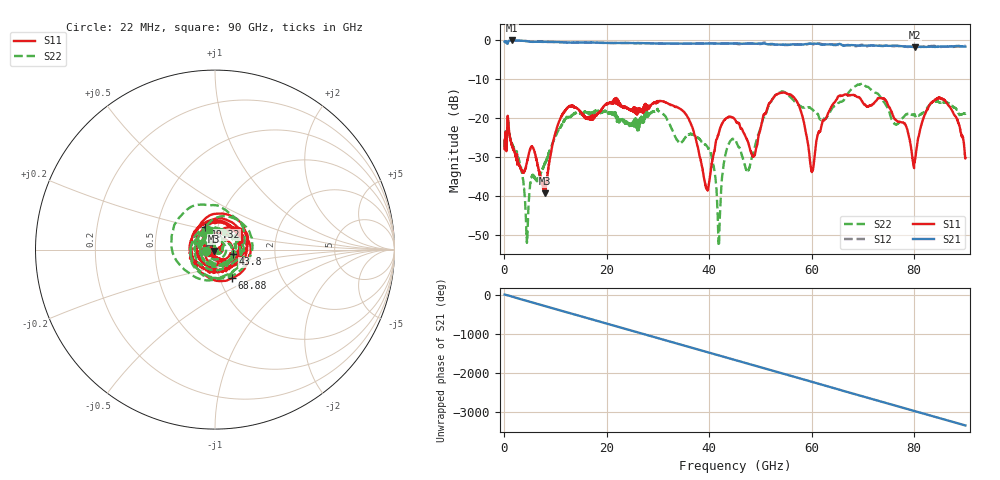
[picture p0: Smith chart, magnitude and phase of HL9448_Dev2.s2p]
! 5/9/2022 12:37:12 PM
! C:\USERS\VECTORSTARUSER\DESKTOP\JASON\HL9449-11\HL9449-11-NE04.S2P
! CHANNEL.1
! TR.MEASUREMENT
! CORRECTED.DATA
# GHZ S RI R 50.0
! FREQ.GHZ  S11RE  S11IM  S21RE  S21IM  S12RE  S12IM  S22RE  S22IM
!; PortSelection: Port_12
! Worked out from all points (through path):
!   4091 points, 22 MHz to 90 GHz, reference 50 ohm
!   highest |S21| = -0.24 dB at 1.386 GHz (marker M1); lowest = -2.0 dB at 80.15 GHz (marker M2)
!   group delay of S21, straight-line fit = 103 ps
!   lowest |S11| = -39.3 dB at 7.942 GHz (marker M3), VSWR 1.02, Z = 49.2 - j0.693 ohm
!   |S11| at or under -10 dB: start of sweep to end of sweep
!   |S22| runs from -52.9 to -11.3 dB; largest |S21 - S12| = 0.038
!   S11 on the Smith chart (normalised r, x): 22 MHz: 0.90, -0.02; 19.32 GHz: 0.87, +0.22; 43.8 GHz: 1.22, -0.06; 68.88 GHz: 1.14, -0.38; 90 GHz: 0.96, -0.04
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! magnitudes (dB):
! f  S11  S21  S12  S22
! 22 MHz  -25.7  -0.5  -0.5  -25.6
! 1.386 GHz  -26.8  -0.2  -0.2  -26.9
! 4.356 GHz  -31.5  -0.4  -0.4  -51.1
! 7.942 GHz  -39.3  -0.6  -0.6  -31.8
! 11.09 GHz  -19.7  -0.7  -0.7  -22.2
! 15.03 GHz  -18.8  -0.8  -0.8  -19.1
! 19.32 GHz  -17.2  -0.9  -0.9  -18.5
! 30.03 GHz  -15.8  -1.0  -1.0  -18.3
! 35.77 GHz  -19.9  -1.1  -1.0  -24.5
! 39.51 GHz  -37.9  -1.0  -1.0  -27.3
! 41.84 GHz  -24.0  -1.1  -1.0  -52.2
! 43.8 GHz  -19.8  -1.0  -1.0  -26.7
! 45.01 GHz  -20.5  -1.0  -1.0  -25.6
! 48.6 GHz  -29.9  -1.1  -1.0  -28.9
! 56.1 GHz  -14.4  -1.3  -1.3  -15.1
! 60.02 GHz  -33.9  -1.1  -1.1  -17.8
! 63.98 GHz  -16.9  -1.3  -1.2  -17.6
! 68.88 GHz  -14.7  -1.5  -1.7  -11.6
! 75.02 GHz  -17.2  -1.6  -1.6  -18.1
! 80.15 GHz  -31.0  -2.0  -1.7  -19.4
! 84.81 GHz  -14.9  -1.8  -1.9  -16.0
! 90 GHz  -30.4  -1.8  -1.6  -18.9
